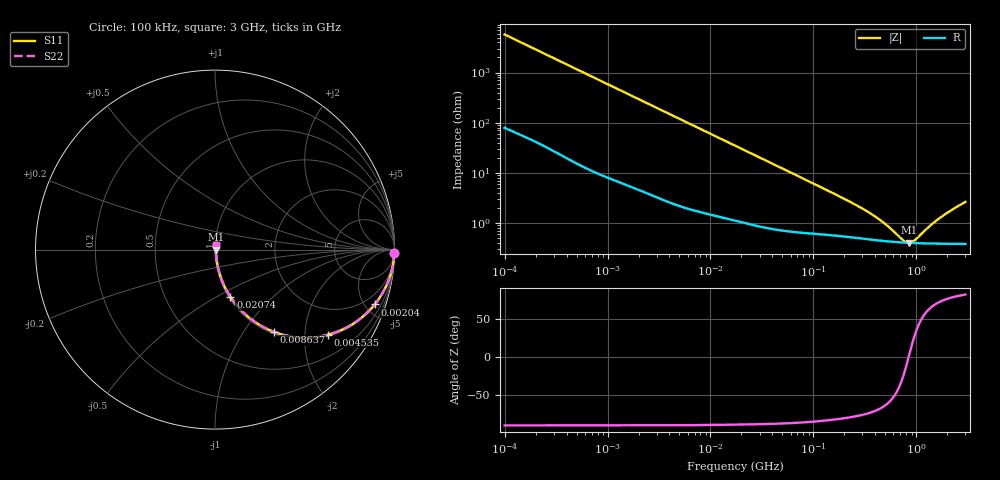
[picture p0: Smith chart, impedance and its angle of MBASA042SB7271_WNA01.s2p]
! MBASA042SB7271_WNA01  S-PARAMETER MODEL  ( Standard Model )
! Model Generated by TAIYO YUDEN Corporation (https://www.yuden.co.jp/en/)
! Version 1.0
! TAIYO YUDEN Control No. 250312
! Copyright(c) 2025 TAIYO YUDEN CO.,LTD. All Rights Reserved.
! Product Description (link to TY-COMPAS)
! https://ds.yuden.co.jp/TYCOMPAS/or/detail?pn=MBASA042SB7271KWNA01&u=M
! Products Name : Multilayer Ceramic Capacitors
! Characteristics :
!  Capacitance : 270 [pF] , Rated Voltage : 4 [V] , TCC : X7R
!  Case Size : 0.4 x 0.2 / 0.016 x 0.008 [mm/inch] , Thickness : 0.2 / 0.008 [mm/inch]
!  (Conditions: Temperature = 25 [degC] , DC Bias Voltage = 0 [V])
! External Node Assignments :
!  1  o---| |---o  2
! GND o---------o GND
! Frequency Range : 100kHz  -  3GHz  [ 401 STEP ]
# MHZ S RI R 50
! Freq[MHz].  S11 Real  S11 Imag  S21 Real  S21 Imag  S12 Real  S12 Imag  S22 Real  S22 Imag
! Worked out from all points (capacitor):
!   401 points, 100 kHz to 3 GHz, reference 50 ohm
!   read as one part in series: C = 276 pF near 105.3 kHz
!   lowest |Z| = 400 mohm at 848.5 MHz (marker M1)
!   series resonance near 842.2 MHz, so ESL is about 130 pH
!   S11 on the Smith chart (normalised r, x): 100 kHz: open; 2.04 MHz: 1.09, -5.79; 4.535 MHz: 1.05, -2.62; 8.637 MHz: 1.03, -1.38; 20.74 MHz: 1.02, -0.58; 3 GHz: 1.01, +0.05
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0.1  0.9995 -0.0173  0.000539 0.0173  0.000539 0.0173  0.9995 -0.0173
0.562235  0.9896 -0.095  0.0104 0.095  0.0104 0.095  0.9896 -0.095
1.18716  0.9583 -0.193  0.0417 0.193  0.0417 0.193  0.9583 -0.193
2.039661  0.8897 -0.3056  0.1103 0.3056  0.1103 0.3056  0.8897 -0.3056
3.161081  0.775 -0.4095  0.225 0.4095  0.225 0.4095  0.775 -0.4095
4.534557  0.6301 -0.474  0.3699 0.474  0.3699 0.474  0.6301 -0.474
6.178009  0.4825 -0.49  0.5175 0.49  0.5175 0.49  0.4825 -0.49
8.636841  0.3276 -0.4581  0.6724 0.4581  0.6724 0.4581  0.3276 -0.4581
12.38951  0.1965 -0.384  0.8035 0.384  0.8035 0.384  0.1965 -0.384
17.7727  0.1108 -0.2982  0.8892 0.2982  0.8892 0.2982  0.1108 -0.2982
20.74485  0.0859 -0.2634  0.9141 0.2634  0.9141 0.2634  0.0859 -0.2634
42.68829  0.0267 -0.1375  0.9733 0.1375  0.9733 0.1375  0.0267 -0.1375
97.38194  0.00987 -0.0614  0.9901 0.0614  0.9901 0.0614  0.00987 -0.0614
302.6647  0.00515 -0.0183  0.9949 0.0183  0.9949 0.0183  0.00515 -0.0183
423.1245  0.00458 -0.0114  0.9954 0.0114  0.9954 0.0114  0.00458 -0.0114
547.5153  0.00427 -0.00685  0.9957 0.00685  0.9957 0.00685  0.00427 -0.00685
745.9503  0.00404 -0.00189  0.996 0.00189  0.996 0.00189  0.00404 -0.00189
848.5431  0.00398 0.000118  0.996 -0.000118  0.996 -0.000118  0.00398 0.000118
965.2458  0.00394 0.00214  0.9961 -0.00214  0.9961 -0.00214  0.00394 0.00214
1349.411  0.00392 0.00766  0.9961 -0.00766  0.9961 -0.00766  0.00392 0.00766
1746.113  0.00398 0.0125  0.996 -0.0125  0.996 -0.0125  0.00398 0.0125
3000  0.00445 0.0257  0.9955 -0.0257  0.9955 -0.0257  0.00445 0.0257
